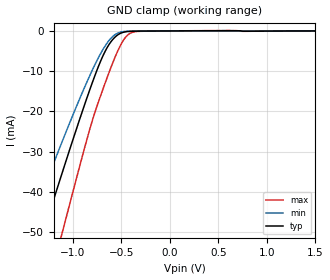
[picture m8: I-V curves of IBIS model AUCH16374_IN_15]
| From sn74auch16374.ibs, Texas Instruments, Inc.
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[Model]   AUCH16374_IN_15
Model_type  Input
Vinl=0.49
Vinh=1.04
| variable   typ   min   max
C_comp   2.77pF   2.17pF   3.17pF
[Temperature Range]   40   100   -40
| Ambient temperature   25   85   -40
[Voltage range]   1.5   1.4   1.6
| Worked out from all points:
|   GND clamp passes 1 mA (typ) near -0.54 V on its own axis
[GND Clamp]
| AUCH16374_IN_15
|   Voltage   I(typ)   I(min)   I(max)
-3.6V     -229mA     -190.7mA   -276.9mA
-1.46V    -61.9mA    -49.16mA   -82.33mA
-1.325V   -51.51mA   -40.65mA   -69.89mA
-1.285V   -48.44mA   -38.15mA   -66.2mA
-1.12V    -35.93mA   -28.02mA   -50.98mA
-1.07V    -32.18mA   -25.01mA   -46.37mA
-810mV    -13.5mA    -10.24mA   -23.06mA
-690mV    -6.161mA   -4.594mA   -14.42mA
-570mV    -1.632mA   -991.7uA   -6.761mA
-430mV    -139.2uA   -76.04uA   -919.2uA
-305mV    -44.78uA   -28.24uA   -92.97uA
1.5V      189.6pA    533.5nA    87.79pA
